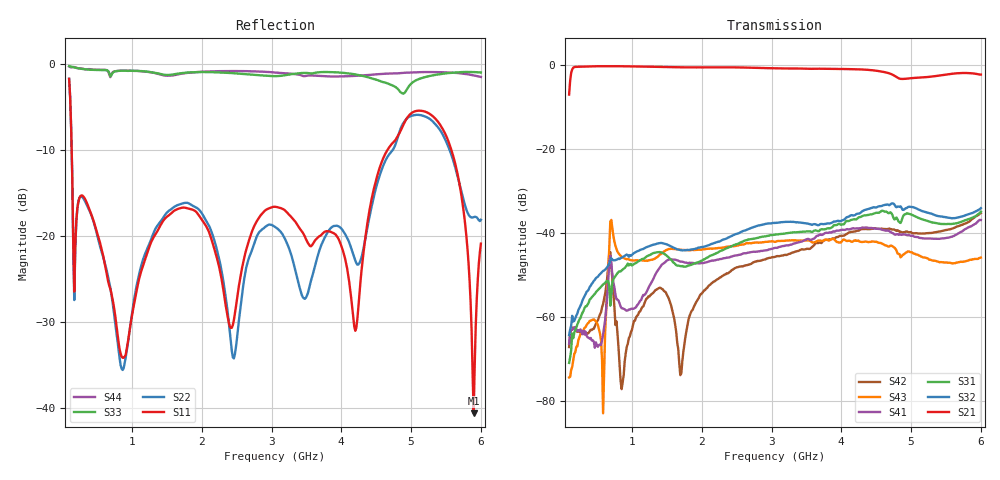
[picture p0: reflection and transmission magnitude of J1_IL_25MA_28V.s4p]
!Keysight Technologies,N5242B,MY61256241,Z.15.82.127
!Date: Friday, August 25, 2023 02:14:11
!Correction: S11(C  4-Port  )
!S12(C  4-Port  )
!S13(C  4-Port  )
!S14(C  4-Port  )
!S21(C  4-Port  )
!S22(C  4-Port  )
!S23(C  4-Port  )
!S24(C  4-Port  )
!S31(C  4-Port  )
!S32(C  4-Port  )
!S33(C  4-Port  )
!S34(C  4-Port  )
!S41(C  4-Port  )
!S42(C  4-Port  )
!S43(C  4-Port  )
!S44(C  4-Port  )
!S4P File: Measurements: <S11,S12,S13,S14>,
!<S21,S22,S23,S24>,
!<S31,S32,S33,S34>,
!<S41,S42,S43,S44>:
# Hz S  dB  R 50
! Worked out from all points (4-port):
!   401 points, 100 MHz to 6 GHz, reference 50 ohm
!   strongest paths, dB at 100 MHz, 1.575 GHz, 3.05 GHz, 4.525 GHz, 6 GHz:
!     S21: -7.1, -0.6, -0.9, -1.5, -2.3
!     S32: -64.4, -43.4, -37.6, -33.8, -34.1
!     S31: -71.0, -46.7, -40.5, -35.3, -35.0
!     S41: -66.5, -46.3, -43.6, -39.1, -37.0
!     S43: -74.4, -43.8, -42.2, -42.3, -45.9
!     S42: -67.2, -58.3, -45.7, -39.1, -35.3
!   lowest |S11| = -40.7 dB at 5.897 GHz (marker M1), VSWR 1.02, Z = 49.6 + j0.816 ohm
!   |S11| at or under -10 dB: 136.5 MHz to 4.661 GHz (4.525 GHz wide, 189 % of centre); 5.577 GHz to end of sweep
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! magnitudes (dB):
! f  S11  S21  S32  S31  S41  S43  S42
! 100 MHz  -1.7  -7.1  -64.4  -71.0  -66.5  -74.4  -67.2
! 586.8 MHz  -22.3  -0.3  -49.1  -52.3  -64.2  -83.0  -57.0
! 719.5 MHz  -27.3  -0.4  -46.4  -51.8  -49.9  -39.0  -51.5
! 867 MHz  -34.2  -0.4  -45.8  -48.8  -58.0  -45.9  -75.5
! 5.159 GHz  -5.5  -3.0  -34.8  -36.8  -41.3  -45.8  -40.2
! 5.897 GHz  -40.7  -2.1  -35.2  -36.3  -38.1  -46.3  -36.5
! 6 GHz  -20.9  -2.3  -34.1  -35.0  -37.0  -45.9  -35.3
